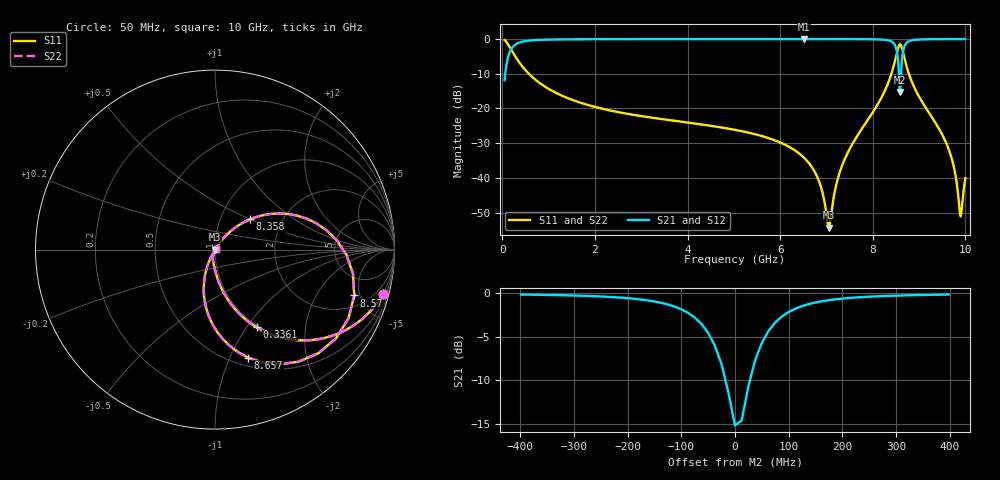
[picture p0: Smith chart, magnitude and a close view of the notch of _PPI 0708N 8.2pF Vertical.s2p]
! S-Parameter data specifications (vertical orientation):
! Substrate: 40-mil Rogers 3003C, Substrate thickness, H=1.016mm, Dielectric constant, Er=3, Conductor thickness, T_mtl=0.043mm, Loss Tangent, Tand=0.003
! PCB Mounting Pad Footprint: Pad width, PadW=2.54mm , Pad length, PadL=0.51mm , Pad gap, PadG (edge-to-edge)=0.71mm , Reference planes=1.73mm apart
! Created Tue Jan 16 08:46:41 2018
# GHz S MA R 50
! 2 Port Network Data from SP1.SP block
! freq  magS11  angS11  magS21  angS21  magS12  angS12  magS22  angS22
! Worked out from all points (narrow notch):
!   801 points, 50 MHz to 10 GHz, reference 50 ohm
!   highest |S21| = -0.02 dB at 6.518 GHz (marker M1); lowest = -15.2 dB at 8.582 GHz (marker M2)
!   notch at M2: 15.2 dB deep, 66.5 MHz wide at half that depth
!   lowest |S11| = -54.3 dB at 7.052 GHz (marker M3), VSWR 1.00, Z = 50.2 - j0.0892 ohm
!   |S11| at or under -10 dB: 573.6 MHz to 8.403 GHz (7.829 GHz wide, 174 % of centre); 8.779 GHz to end of sweep
!   |S22| runs from -54.3 to -0.3 dB; largest |S21 - S12| = 0
!   S11 on the Smith chart (normalised r, x): 50 MHz: 0.98, -7.48; 336.1 MHz: 0.98, -1.12; 8.358 GHz: 1.38, +0.50; 8.57 GHz: 2.88, -4.42; 8.657 GHz: 0.59, -1.17; 10 GHz: 1.02, +0.01
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0.05  0.9668 -15.0  0.2554 75.0  0.2554 75.0  0.9668 -15.0
0.1619375  0.7599 -41.1  0.6498 48.9  0.6498 48.9  0.7599 -41.1
0.3360625  0.4919 -61.8  0.8703 28.2  0.8703 28.2  0.4919 -61.8
0.8833125  0.2145 -80.8  0.9763 9.1  0.9763 9.1  0.2145 -80.8
1.716625  0.1193 -89.3  0.9923 0.5  0.9923 0.5  0.1193 -89.3
3.370812  0.07146 -97.8  0.9966 -8.4  0.9966 -8.4  0.07146 -97.8
5.025  0.04925 -104.4  0.9975 -15.6  0.9975 -15.6  0.04925 -104.4
6.5175  0.01949 -108.1  0.998 -22.6  0.998 -22.6  0.01949 -108.1
6.691625  0.01409 -106.9  0.998 -23.6  0.998 -23.6  0.01409 -106.9
6.878188  0.007529 -101.0  0.9979 -24.6  0.9979 -24.6  0.007529 -101.0
7.052313  0.001923 -27.5  0.9978 -25.6  0.9978 -25.6  0.001923 -27.5
7.388125  0.01822 54.8  0.9972 -27.8  0.9972 -27.8  0.01822 54.8
8.345812  0.2455 41.8  0.9521 -44.3  0.9521 -44.3  0.2455 41.8
8.35825  0.2585 40.8  0.9473 -45.1  0.9473 -45.1  0.2585 40.8
8.482625  0.4942 22.5  0.8063 -59.9  0.8063 -59.9  0.4942 22.5
8.569688  0.8168 -18.2  0.2697 -72.2  0.2697 -72.2  0.8168 -18.2
8.582125  0.8366 -27.2  0.1733 -49.0  0.1733 -49.0  0.8366 -27.2
8.65675  0.63 -72.9  0.6756 7.3  0.6756 7.3  0.63 -72.9
8.806  0.2811 -102.1  0.9437 -15.3  0.9437 -15.3  0.2811 -102.1
9.626875  0.02722 -117.1  0.9965 -32.8  0.9965 -32.8  0.02722 -117.1
9.888063  0.002889 -51.9  0.9968 -35.2  0.9968 -35.2  0.002889 -51.9
10  0.009896 37.2  0.9967 -36.2  0.9967 -36.2  0.009896 37.2
